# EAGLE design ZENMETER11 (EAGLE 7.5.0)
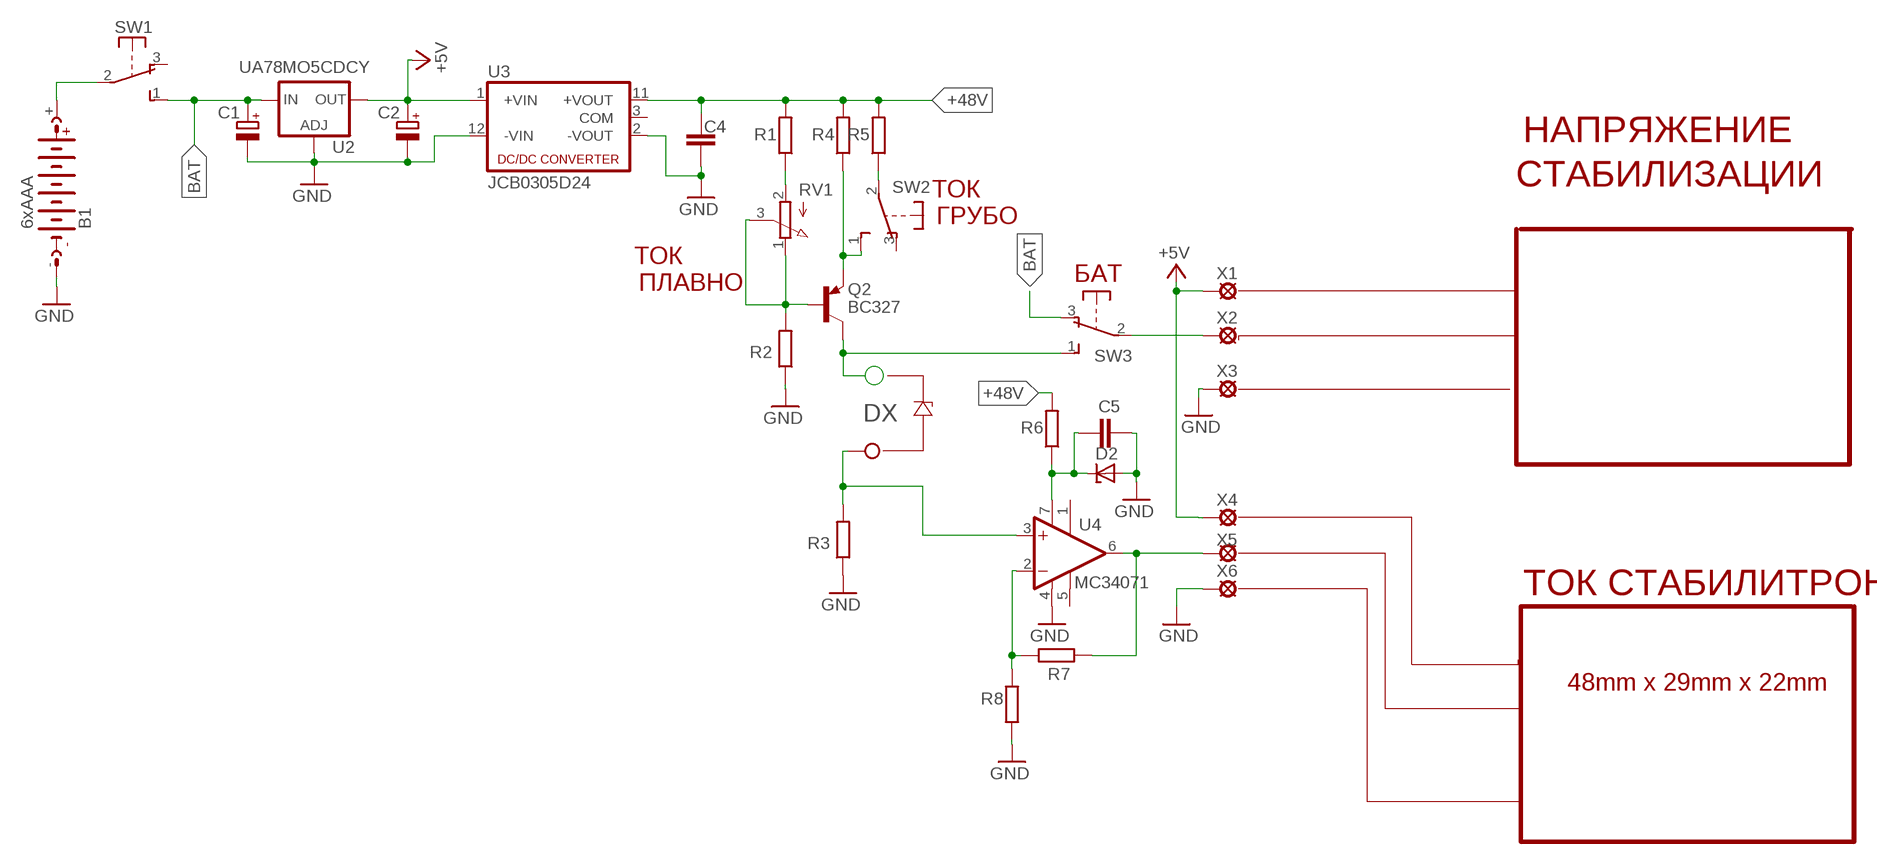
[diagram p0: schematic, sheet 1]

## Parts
B1  6xAAA  AB9V  [AB9V]
C1  CPOL-EUE2.5-6  [E2,5-6]
C2  CPOL-EUE2.5-6  [E2,5-6]
C4  C-EUC1206  [C1206]
C5  C-EUC1206  [C1206]
D2  1N4755A  1N4728  [DO41Z10]
DX  TPPAD1-20Y  [P1-20Y]
Q2  BC327  [TO92]
R1  R-EU_R1206  [R1206]
R2  R-EU_R1206  [R1206]
R3  R-EU_R1206  [R1206]
R4  R-EU_R1206  [R1206]
R5  R-EU_R1206  [R1206]
R6  R-EU_R1206  [R1206]
R7  R-EU_R1206  [R1206]
R8  R-EU_R1206  [R1206]
RV1  PTV09A2  [PTV09A2]
SW1  9077-1  [9077-1]
SW2  9077-1  [9077-1]
SW3  9077-1  [9077-1]
U2  UA78MO5CDCY  LD117AS33TR  [SOT223]
U3  JCB0305D24  [JCB0305D24]
U4  MC34071  OPA131U  [SO08]
X1  LSP10  [LSP10]
X2  LSP10  [LSP10]
X3  LSP10  [LSP10]
X4  LSP10  [LSP10]
X5  LSP10  [LSP10]
X6  LSP10  [LSP10]

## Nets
+5V: C2.+ U2.3(OUT) U3.1(+VIN) X1.MP X4.MP
+48V: C4.2 R1.2 R4.2 R5.2 R6.2 U3.11(+VOUT)
BAT: C1.+ SW1.1(S) SW3.3(O) U2.1(IN)
GND: B1.- C1.- C2.- C4.1 C5.1 D2.A R2.1 R3.1 R8.2 U2.2(ADJ) U3.2(-VOUT) U3.12(-VIN) U4.4(V-) X3.MP X6.MP
GND1: DX.TP R3.2 U4.3(+IN)
N$1: SW3.2(P) X2.MP
N$2: Q2.2(B) R2.2 RV1.1(E) RV1.3(S)
N$3: R1.1 RV1.2(A)
N$4: Q2.1(E) R4.1 SW2.1(S)
N$5: Q2.3(C) SW3.1(S)
N$6: R5.1 SW2.2(P)
N$7: C5.2 D2.C R6.1 U4.7(V+)
N$9: R7.1 U4.6(OUT) X5.MP
N$10: R7.2 R8.1 U4.2(-IN)
N$41: B1.+ SW1.2(P)
Unconnected: SW1.3(O) SW2.3(O) U3.3(COM) U4.1(TRIM1) U4.5(TRIM2)

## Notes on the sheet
- НАПРЯЖЕНИЕ
- СТАБИЛИЗАЦИИ
- ТОК
- ГРУБО
- ТОК
- БАТ
- ПЛАВНО
- ТОК СТАБИЛИТРОНА
- 48mm x 29mm x 22mm

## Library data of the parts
B1 = battery:AB9V: 9-V BATTERY CLIP
C1 C2 = rcl:CPOL-EU: POLARIZED CAPACITOR, European symbol
C4 C5 = rcl:C-EU: CAPACITOR, European symbol
D2 = diode:1N4728: Z DIODE
DX = testpad:TP: Test pad
Q2 = transistor-pnp:BC327: PNP Transistor
R1-R8 = rcl:R-EU_: RESISTOR, European symbol
RV1 = pot:PTV09A2
SW1-SW3 = switch-misc:9077-1: MARQUARDT SWITCH 9077.0100 Distributor: Buerklin
U2 = v-reg:LD117A?*: Low drop fixed and adjustable positive voltage regulators 1 A Source: http://www.st.com/stonline/products/literature/ds/7194/ld1117axx.pdf
U3 = dc-dc-converter:JCB0305D24: Isolated Board Mount DC/DC Converter, 2:1 Input, ITE, 2 Output, 3 W, 24 V, 63 mA, -24 V
U4 = burr-brown:OPA131: Operational Amplifiers General Purpose FET-Input; MF: TEXAS INSTRUMENT CONNECTORS; MPN: OPA131U; OC_FARNELL: 1459547; OC_NEWARK: 75C4591
X1-X6 = solpad:LSP10: SOLDER PAD

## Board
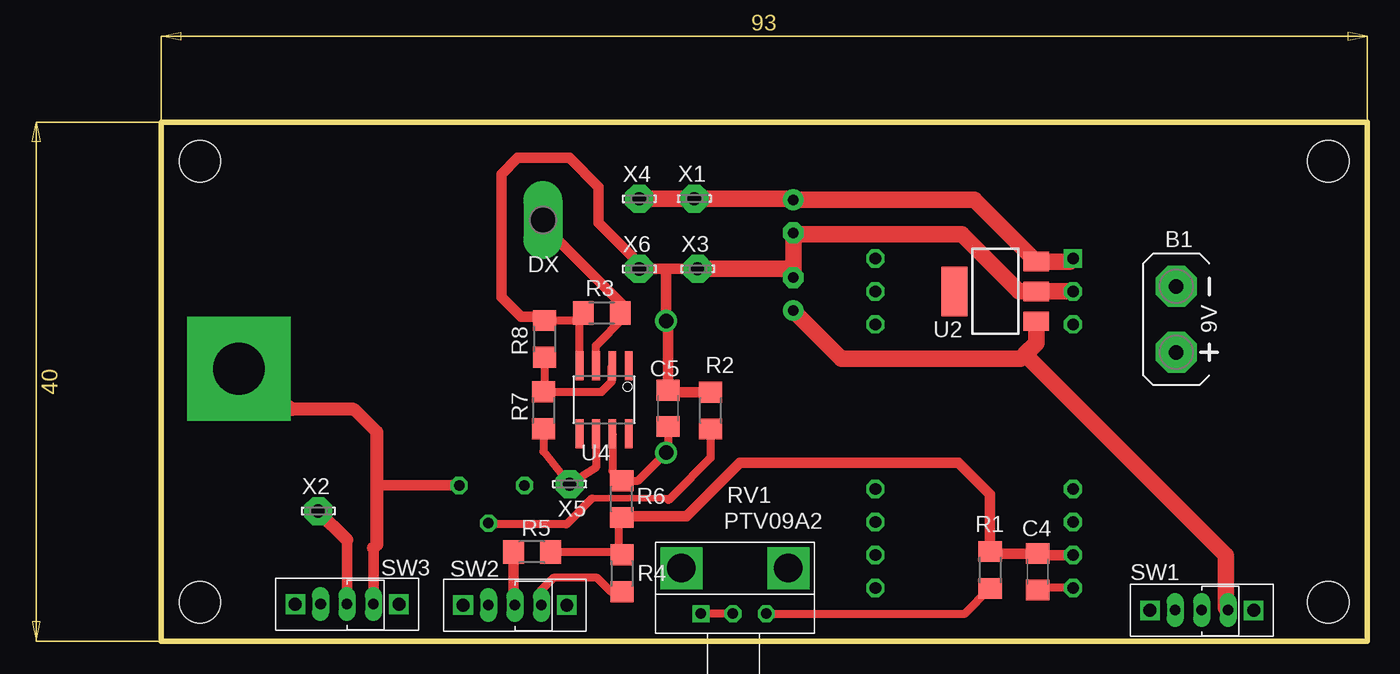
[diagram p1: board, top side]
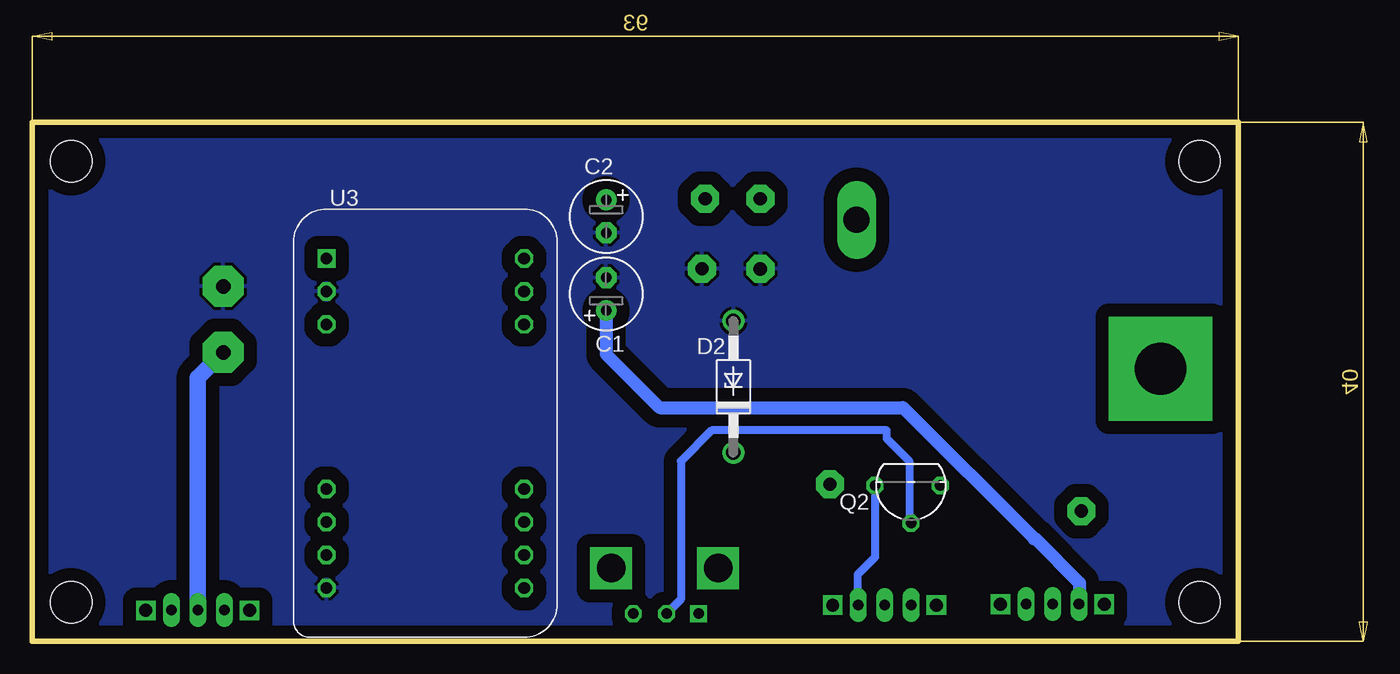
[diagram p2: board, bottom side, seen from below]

Size 102.92 x 46.92 mm. Coordinates in mm from the lower left corner, seen from the top.
Outline: 9.93,0 9.93,40 102.92,40 102.92,0 9.93,0
Copper layers (1*16): Top 0.035mm / dielectric 1.5mm / Bottom 0.035mm
Design rules "default": minimum track width 10mil, minimum drill 24mil, track to track 8mil, track to pad 8mil, pad to pad 8mil, via to via 8mil, smd to smd 8mil, copper to edge 40mil, drill to drill 8mil, minimum pad ring 10mil, minimum via ring 8mil, stop-mask expansion 4mil, vias tented up to drill 0mil, thermal gap 10mil
Holes 3.2 mm at 99.92,37 99.92,3 12.93,3 12.93,37

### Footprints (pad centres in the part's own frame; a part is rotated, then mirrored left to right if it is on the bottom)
AB9V = drill 1.118 pad 3.15 octagon: + 0,2.54; - 0,-2.54
E2,5-6 = drill 0.813 pad 1.6: + -1.27,0 | drill 0.813 pad 1.6 octagon: - 1.27,0
C1206 = smd 1.6 x 1.8: 1 -1.4,0; 2 1.4,0
DO41Z10 = drill 1.118: A 5.08,0; C -5.08,0
P1-20Y = drill 2.007 pad 2.54 long: TP 0,0
TO92 = drill 0.813 octagon: 1 2.77,0; 2 0,2.905; 3 -2.27,0
R1206 = smd 1.6 x 1.803: 1 -1.422,0; 2 1.422,0
PTV09A2 = drill 0.8 square: 1 0,0 | drill 0.8 octagon: 2 5.04,0; 3 2.46,0 | drill 2.2 square: P$1 -1.5,3.5; P$2 6.75,3.5
9077-1 = drill 0.813 long: 1 -2.04,-1.016; 2 0,-1.016; 3 2.04,-1.016 | drill 1 square: P$1 -4,-1; P$2 4,-1
SOT223 = smd 1.5 x 2: 1 -2.3,-3.15; 2 0,-3.15; 3 2.3,-3.15 | smd 3.8 x 2: 4 0,3.15
JCB0305D24 = drill 0.9 square: 1 0,0 | drill 0.9 octagon: 2 2.54,0; 3 5.08,0; 9 17.78,0; 10 20.32,0; 11 22.86,0; 12 25.4,0; 13 25.4,15.24; 14 22.86,15.24; 15 20.32,15.24; 16 17.78,15.24; 22 5.08,15.24; 23 2.54,15.24; P$8 0,15.24
SO08 = smd 0.61 x 2.21: 1 -1.905,-2.616; 2 -0.635,-2.616; 3 0.635,-2.616; 4 1.905,-2.616; 5 1.905,2.616; 6 0.635,2.616; 7 -0.635,2.616; 8 -1.905,2.616
LSP10 = drill 1.016 pad 2.159 octagon: MP 0,0

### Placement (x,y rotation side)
B1  88.2,24.81 180 top
C1  58.67,26.75 90 bottom
C2  58.67,32.75 270 bottom
C4  77.52,5.35 90 top
C5  49.02,17.95 270 top
D2  48.86,19.61 90 bottom
DX  39.38,32.47 180 top
Q2  35.17,12 180 bottom
R1  73.84,5.48 90 top
R2  52.3,17.77 270 top
R3  43.91,25.29 0 top
R4  45.47,5.23 90 top
R5  38.53,6.88 0 top
R6  45.45,10.95 270 top
R7  39.41,17.8 90 top
R8  39.5,23.3 90 top
RV1  51.55,2.12 0 top
SW1  90.17,1.38 180 top
SW2  37.21,1.77 180 top
SW3  24.27,1.84 180 top
U2  74.25,26.96 90 top
U3  80.24,29.5 270 bottom
U4  44.08,18.61 180 top
X1  51.05,34.11 0 top
X2  22.05,10.03 0 top
X3  51.3,28.7 0 top
X4  46.8,34.1 0 top
X5  41.43,12.11 180 top
X6  46.8,28.69 0 top

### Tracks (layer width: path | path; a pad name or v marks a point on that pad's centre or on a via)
+5V
  Top 1.27: X4.MP X1.MP 58.58,34.11 C2.+ 72.64,34.02 U2.3 80,29.26 U3.1
+48V
  Top 0.61: R5.2 44.92,6.88 45.24,6.88 | 45.24,6.88 R4.2 | 45.24,6.88 45.24,9.32 R6.2 | 80.38,6.5 U3.11
  Top 0.813: U3.11 77.62,6.64 C4.2 74,6.75 R1.2 73.84,11.33 71.42,13.75 54.55,13.75 50.42,9.62 45.54,9.62 R6.2 | 44.93,6.88 44.92,6.88
BAT
  Top 1.27: U2.1 77.41,22.98 76.55,22.12 | 76.55,22.12 76.17,21.75 62.41,21.75 C1.+ | 76.55,22.12 92.05,6.62 92.05,2.56 SW1.1
  Bottom 1.016: C1.+ 58.67,22.12 54.55,18 35.8,18 25.68,7.88 25.55,7.88 22.18,4.5 22.18,2.91 SW3.3
GND
  Top 0.61: U4.4 42.18,24.75 | 42.18,24.75 42.18,24.99 R3.1 | R8.2 42.15,24.72 42.18,24.75 | U3.12 77.66,4.1 C4.1
  Top 0.813: R8.2 39.22,25 37.67,25 36.17,26.5 36.17,36 37.42,37.25 41.42,37.25 43.67,35 43.67,32.25 46.8,29.13 X6.MP 48.92,28.69 | 48.92,28.69 X3.MP | 48.92,28.69 48.86,28.63 D2.A 49.02,24.54 C5.1 49.17,19.19 R2.1
  Top 1.27: U3.2 U2.2 76.09,26.96 71.67,31.38 58.78,31.38 C2.- 58.67,28.75 | C1.- 58.67,28.75 | X3.MP 58.62,28.7 58.67,28.75
  pour Bottom (isolate 1.016): 10.43,39.62 102.17,39.38 102.17,0.38 10.43,0.62
GND1
  Top 0.61: U4.3 43.45,22.77 45.67,25 45.62,25 R3.2
  Top 0.813: DX.TP 39.38,32.05 45.42,26 45.42,25.39 R3.2
N$1
  Top 0.813: 24.27,7.81 SW3.2
  Top 1.016: 24.27,7.81 X2.MP
N$2
  Top 0.5: 43.17,11 49.17,11 49.36,11.19
  Top 0.61: RV1.3 RV1.1 | R2.2 52.3,14.12 49.36,11.19 49.05,10.88 | 43.17,11 41.17,9 35.27,9 Q2.2
  Bottom 0.61: RV1.3 52.92,3.21 52.92,13.88 50.55,16.25 37.05,16.25 37.05,15.62 35.3,13.88 35.3,9.22 Q2.2
N$3
  Top 0.61: RV1.2 71.91,2.12 R1.1
N$4
  Top 0.61: R4.1 44.62,3.81 43.55,4.88 40.17,4.88 39.17,3.88 39.17,2.86 SW2.1
  Bottom 0.61: 39.17,2.86 SW2.1 39.3,2.84 39.3,5.12 37.95,6.48 Q2.1
N$5  (via drill 4 pad 8)
  Top 0.813: 26.3,7.19 SW3.1 | Q2.3 26.8,12 26.55,12.25
  Top 1.016: v15.93,21 20.05,17.88 24.8,17.88 26.55,16.12 26.55,12.25 26.55,7.43 26.3,7.19
N$6
  Top 0.813: R5.1 37.11,2.89 SW2.2
N$7
  Top 0.61: U4.7 44.72,13.1 R6.1 46.71,12.37 D2.C 49.02,14.68 C5.2
N$9
  Top 0.61: R7.1 39.41,14.62 X5.MP 43.45,13.38 U4.6
N$10
  Top 0.61: U4.2 44.67,21.18 44.67,20 43.9,19.22 R7.2 39.5,19.3 R8.1
N$41
  Bottom 1.27: B1.+ 90.17,20.3 SW1.2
